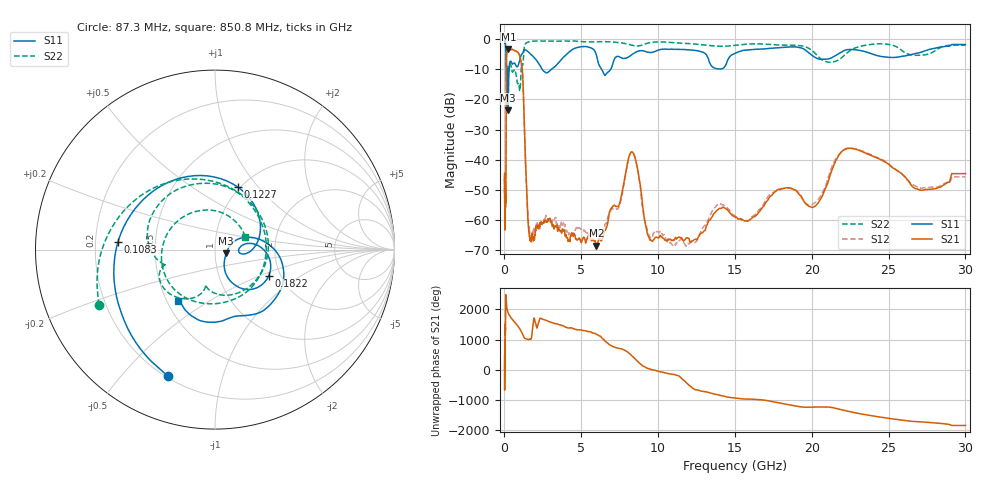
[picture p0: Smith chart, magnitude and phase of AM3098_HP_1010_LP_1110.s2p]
! Date/Time: Thu, Feb 28, 2019 8:42 AM
! Network Analyzer: Agilent Technologies E8364B Rev: A.07.50.67
! Sweep from 0.010 to 30.000 GHz, 1601 Points, Sweep Type: LOG
! Power Supply: 5.023 V, 0.002 A
# Hz S DB R 50
!freq MagS11 AngS11 MagS21 AngS21 MagS12 AngS12 MagS22 AngS22
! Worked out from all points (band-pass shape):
!   1601 points, 10 MHz to 30 GHz, reference 50 ohm
!   highest |S21| = -3.13 dB at 258.6 MHz (marker M1); lowest = -68.7 dB at 5.989 GHz (marker M2)
!   |S21| within 3 dB of the highest: 133.8 MHz to 1.027 GHz (893.6 MHz wide, 154 % of centre)
!   lowest |S11| = -23.6 dB at 241.1 MHz (marker M3), VSWR 1.14, Z = 56.7 - j2.35 ohm
!   |S11| at or under -10 dB: 192.9 MHz to 301.4 MHz (108.5 MHz wide, 43.9 % of centre); 2.472 GHz to 3.034 GHz (562.5 MHz wide, 20.4 % of centre); 6.328 GHz to 6.909 GHz (580.9 MHz wide, 8.78 % of centre)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
!   |S22| runs from -17.1 to -0.5 dB; largest |S21 - S12| = 0.008
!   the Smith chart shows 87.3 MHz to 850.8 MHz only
!   S11 on the Smith chart (normalised r, x): 87.3 MHz: 0.21, -0.67; 108.3 MHz: 0.30, +0.04; 122.7 MHz: 0.97, +0.79; 182.2 MHz: 1.73, -0.58; 850.8 MHz: 0.57, -0.37
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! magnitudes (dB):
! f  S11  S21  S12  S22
! 10 MHz  -0.3  -46.5  -47.2  -0.6
! 38.04 MHz  -0.5  -60.4  -59.1  -1.0
! 87.3 MHz  -2.5  -52.4  -55.1  -2.9
! 108.3 MHz  -5.3  -30.5  -30.4  -6.8
! 122.7 MHz  -8.6  -11.7  -11.7  -10.7
! 144.7 MHz  -17.6  -4.7  -4.7  -13.7
! 182.2 MHz  -9.5  -3.8  -3.8  -9.0
! 241.1 MHz  -23.6  -3.1  -3.1  -10.9
! 258.6 MHz  -18.0  -3.1  -3.1  -10.5
! 550.5 MHz  -8.1  -3.5  -3.4  -10.8
! 850.8 MHz  -9.1  -4.2  -4.2  -14.7
! 1.178 GHz  -4.7  -11.3  -11.2  -8.7
! 1.606 GHz  -4.4  -64.9  -63.1  -0.8
! 2.084 GHz  -6.9  -62.4  -61.3  -0.5
! 5.989 GHz  -5.3  -68.7  -64.2  -0.8
! 7.926 GHz  -6.2  -43.4  -43.9  -1.5
! 8.459 GHz  -4.5  -38.8  -38.8  -2.1
! 9.49 GHz  -4.4  -67.0  -66.0  -1.1
! 10.97 GHz  -3.3  -66.8  -68.6  -1.1
! 20.1 GHz  -5.6  -55.8  -54.8  -4.0
! 22.56 GHz  -3.3  -36.2  -36.3  -3.5
! 30 GHz  -1.7  -44.7  -45.8  -1.9
